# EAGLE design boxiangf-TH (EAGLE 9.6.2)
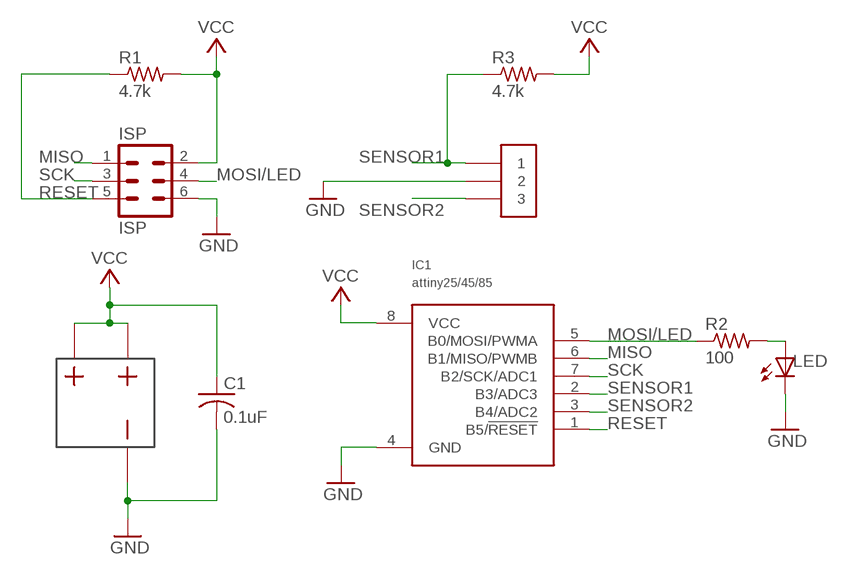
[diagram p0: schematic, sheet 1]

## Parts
C1  0.1uF  CAPACITORTH_CAP  [C025-025X050]
IC1  attiny25/45/85  ATTINY25TH_ATTINY  [DIL08]
ISP  ISP  6PINCON_ISPTH_6PIN  [6P2R0.1IN]
LED  LEDTH_LED  [LED5MM]
R1  4.7k  RESISTORTH_RESISTOR  [0204/7]
R2  100  RESISTORTH_RESISTOR  [0204/7]
R3  4.7k  RESISTORTH_RESISTOR  [0204/7]
SENSE  3PINCONTH_3PIN  [PUSHCON3]
US1  BATTERYTH_BA2032  [BA2032]

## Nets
GND: C1.2 IC1.4(GND) ISP.6 LED.K(C) SENSE.2 US1.P$1
MISO: IC1.6(B1/MISO/PWMB) ISP.1
MOSI/LED: IC1.5(B0/MOSI/PWMA) ISP.4 R2.1
N$2: LED.A R2.2
RESET: IC1.1(B5/!RESET) ISP.5 R1.1
SCK: IC1.7(B2/SCK/ADC1) ISP.3
SENSOR1: IC1.2(B3/ADC3) R3.1 SENSE.1
SENSOR2: IC1.3(B4/ADC2) SENSE.3
VCC: C1.1 IC1.8(VCC) ISP.2 R1.2 R3.2 US1.P$2 US1.P$3

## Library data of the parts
C1 = TinyGadget:CAPACITOR
IC1 = TinyGadget:ATTINY25
ISP = TinyGadget:6PINCON_ISP
LED = TinyGadget:LED
R1-R3 = TinyGadget:RESISTOR
SENSE = TinyGadget:3PINCON
US1 = TinyGadget:BATTERY

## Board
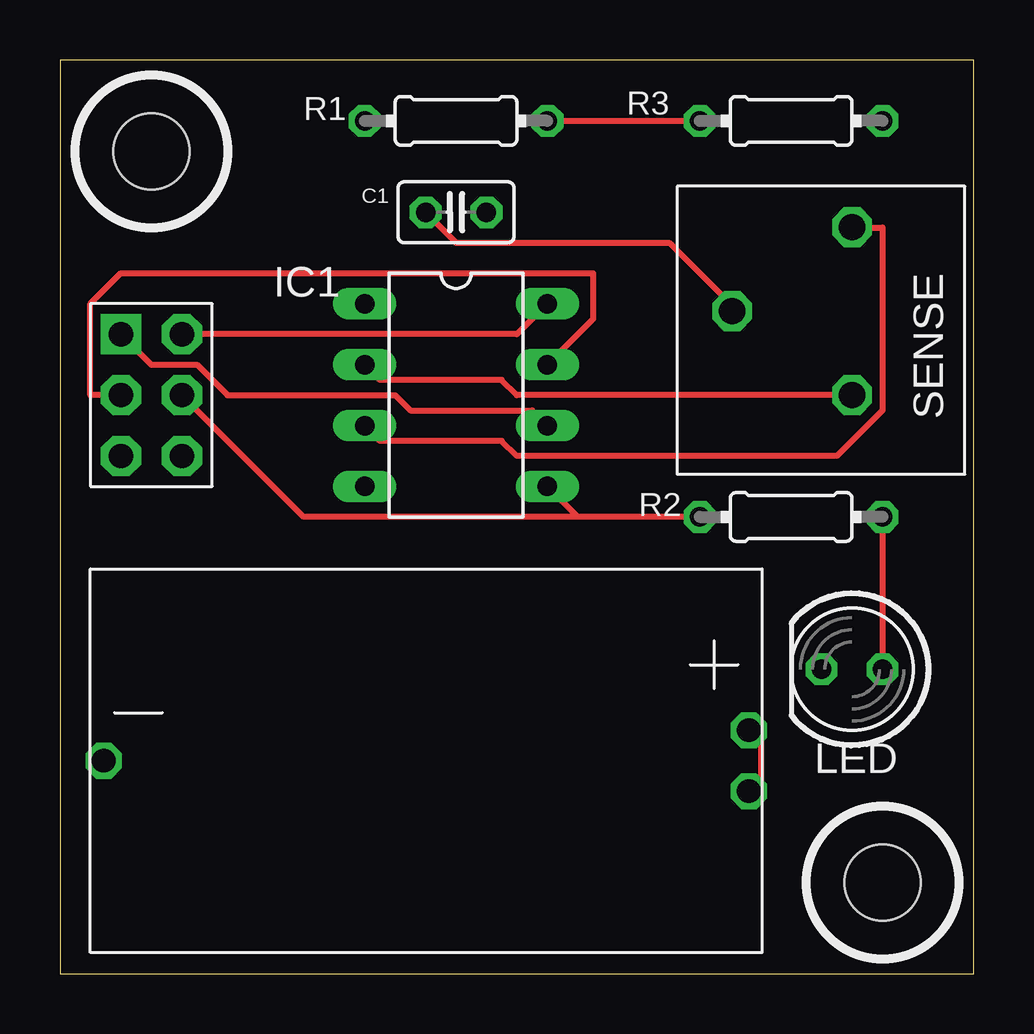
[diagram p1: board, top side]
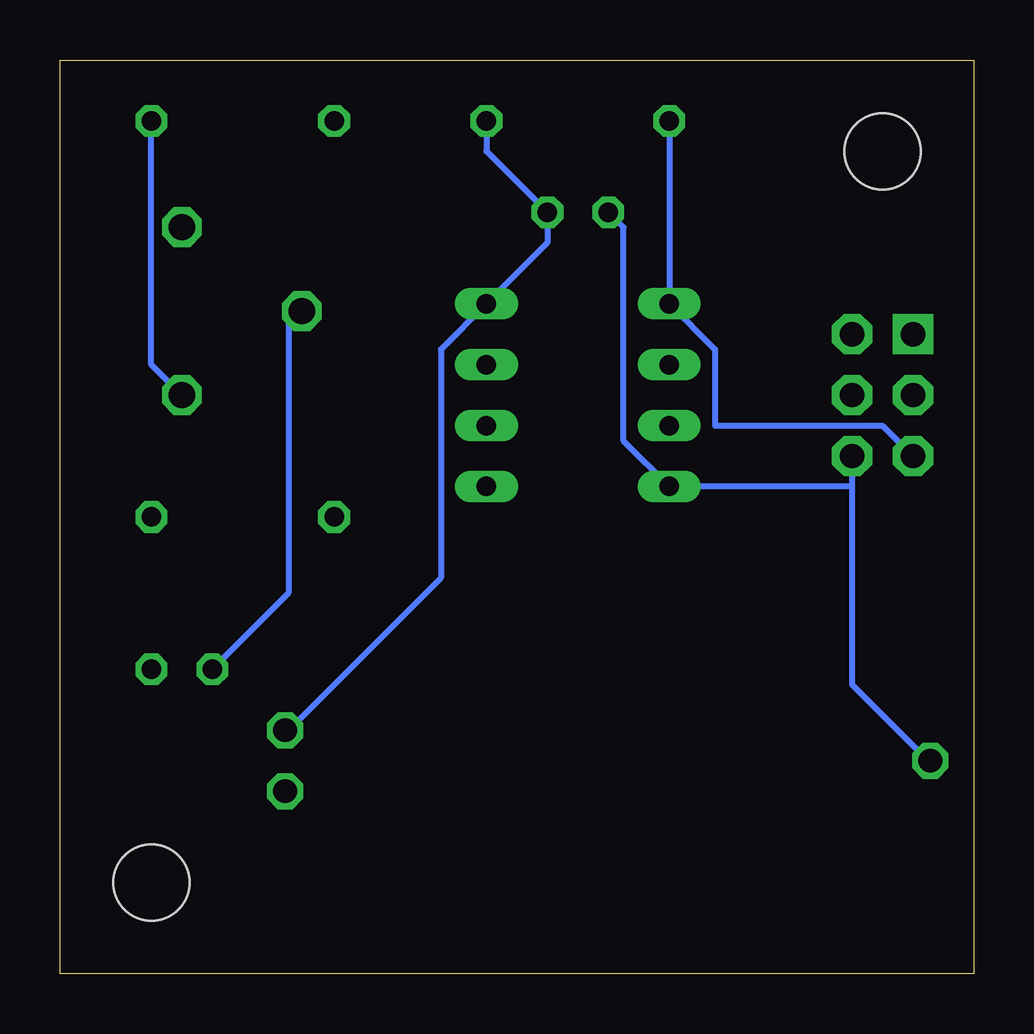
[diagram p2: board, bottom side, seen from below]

Size 38.1 x 38.1 mm. Coordinates in mm from the lower left corner, seen from the top.
Outline: 0,0 38.1,0 38.1,38.1 0,38.1 0,0
Copper layers (1*16): Top 0.035mm / dielectric 1.5mm / Bottom 0.035mm
Design rules "default": minimum track width 6mil, minimum drill 0.35mm, track to track 6mil, track to pad 6mil, pad to pad 6mil, via to via 6mil, smd to smd 6mil, copper to edge 40mil, drill to drill 6mil, minimum pad ring 10mil, minimum via ring 8mil, stop-mask expansion 4mil, vias tented up to drill 0mil, thermal gap 10mil
Holes 3.17 mm at 3.81,34.29 34.29,3.81

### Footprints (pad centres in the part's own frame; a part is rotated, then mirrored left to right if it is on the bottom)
C025-025X050 = drill 0.813 octagon: 1 -1.27,0; 2 1.27,0
DIL08 = drill 0.813 long: 1 -3.81,-3.81; 2 -1.27,-3.81; 3 1.27,-3.81; 4 3.81,-3.81; 5 3.81,3.81; 6 1.27,3.81; 7 -1.27,3.81; 8 -3.81,3.81
6P2R0.1IN = drill 1.016 pad 1.676 square: 1 0,0 | drill 1.016 pad 1.676 octagon: 2 0,2.54; 3 2.54,0; 4 2.54,2.54; 5 5.08,0; 6 5.08,2.54
LED5MM = drill 0.813 octagon: A -1.27,0; K 1.27,0
0204/7 = drill 0.813 octagon: 1 -3.81,0; 2 3.81,0
PUSHCON3 = drill 1.1 octagon: 1 0,0; 2 3.5,5; 3 7,0
BA2032 = drill 0.991 octagon: P$1 0.55,0; P$2 27.45,1.27; P$3 27.45,-1.27

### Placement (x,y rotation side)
C1  16.51,31.75 180 top
IC1  16.51,24.13 270 top
ISP  2.54,26.67 270 top
LED  33.02,12.7 180 top
R1  16.51,35.56 0 top
R2  30.48,19.05 0 top
R3  30.48,35.56 180 top
SENSE  33.02,24.13 90 top
US1  1.27,8.89 0 top

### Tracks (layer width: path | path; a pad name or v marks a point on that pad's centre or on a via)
GND
  Top 0.152: 27.94,27.94 SENSE.2
  Top 0.254: 27.94,27.94 25.4,30.48 16.51,30.48 C1.2
  Bottom 0.152: 28.57,27.3 SENSE.2 | 1.91,8.89 US1.P$1
  Bottom 0.254: LED.K 28.57,15.88 28.57,27.3 | 5.08,20.32 IC1.4 14.61,22.23 14.61,31.11 C1.2 | ISP.6 5.08,20.32 | 1.91,8.89 5.08,12.06 5.08,20.32
MISO
  Top 0.254: IC1.6 19.68,23.5 14.61,23.5 13.97,24.13 6.99,24.13 5.71,25.4 3.81,25.4 ISP.1
MOSI/LED
  Top 0.254: 21.59,19.05 IC1.5 | R2.1 21.59,19.05 | ISP.4 10.16,19.05 21.59,19.05
N$2
  Top 0.254: R2.2 LED.A
RESET
  Bottom 0.254: R1.1 IC1.1 10.79,26.04 10.79,22.86 3.81,22.86 ISP.5
SCK
  Top 0.254: IC1.7 22.23,27.3 22.23,29.21 2.54,29.21 1.27,27.94 1.27,24.13 ISP.3
SENSOR1
  Top 0.254: IC1.2 13.34,24.77 18.41,24.77 19.05,24.13 SENSE.1
  Bottom 0.254: R3.1 34.29,25.4 SENSE.1
SENSOR2
  Top 0.152: 33.02,31.11 SENSE.3
  Top 0.254: IC1.3 13.34,22.23 18.41,22.23 19.05,21.59 32.38,21.59 34.29,23.5 34.29,31.11 33.02,31.11
VCC
  Top 0.254: US1.P$3 29.21,7.62 29.21,10.16 US1.P$2 | R1.2 R3.2 | ISP.2 19.05,26.67 IC1.8
  Bottom 0.254: R1.2 20.32,34.29 C1.1 17.78,30.48 IC1.8 22.23,26.04 22.23,16.51 28.57,10.16 US1.P$2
